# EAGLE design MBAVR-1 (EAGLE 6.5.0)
Minimalistic AVR Board
REV: 123
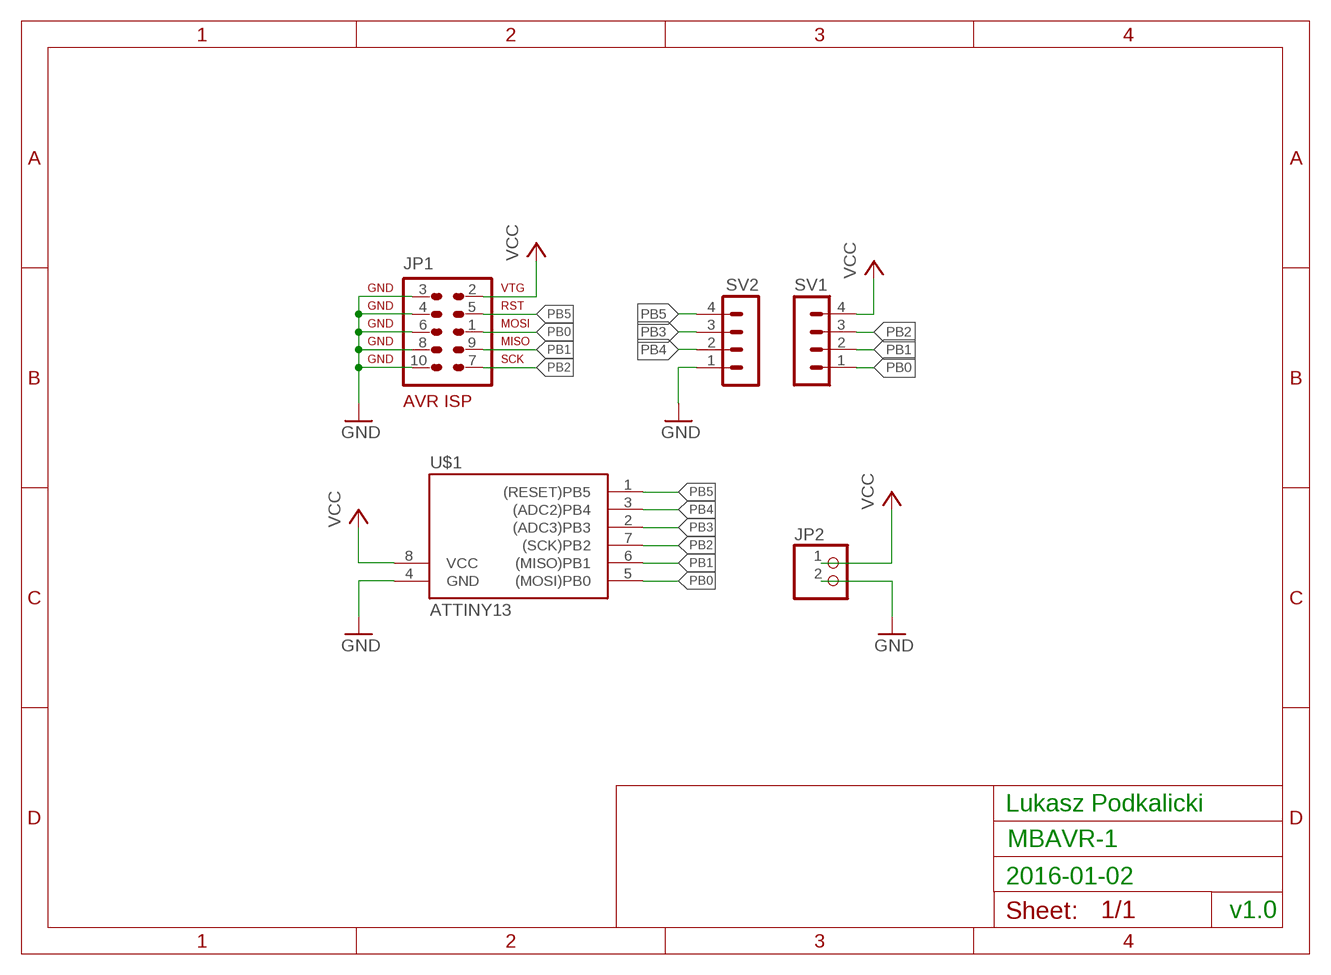
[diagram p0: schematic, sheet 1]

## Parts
JP1  AVR-ISP-10  [AVR-ISP-10]
JP2  PINHD-1X2  [1X02]
SV1  MA04-1  [MA04-1]
SV2  MA04-1  [MA04-1]
U$1  ATTINY13  TINY138P3  [DIL08]

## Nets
GND: JP1.3 JP1.4 JP1.6 JP1.8 JP1.10 JP2.2 SV2.1 U$1.4(GND)
PB0: JP1.1 SV1.1 U$1.5((MOSI)PB0)
PB1: JP1.9 SV1.2 U$1.6((MISO)PB1)
PB2: JP1.7 SV1.3 U$1.7((SCK)PB2)
PB3: SV2.3 U$1.2((ADC3)PB3)
PB4: SV2.2 U$1.3((ADC2)PB4)
PB5: JP1.5 SV2.4 U$1.1((RESET)PB5)
VCC: JP1.2 JP2.1 SV1.4 U$1.8(VCC)

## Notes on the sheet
- Lukasz Podkalicki
- 2016-01-02
- v1.0

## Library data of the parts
JP1 = avr-7:AVR-ISP-10: AVR ISP-10 Serial Programming Header
JP2 = pinhead:PINHD-1X2: PIN HEADER
SV1 SV2 = con-lstb:MA04-1: PIN HEADER; OC_FARNELL: unknown; OC_NEWARK: unknown
U$1 = avr-7:TINY13*

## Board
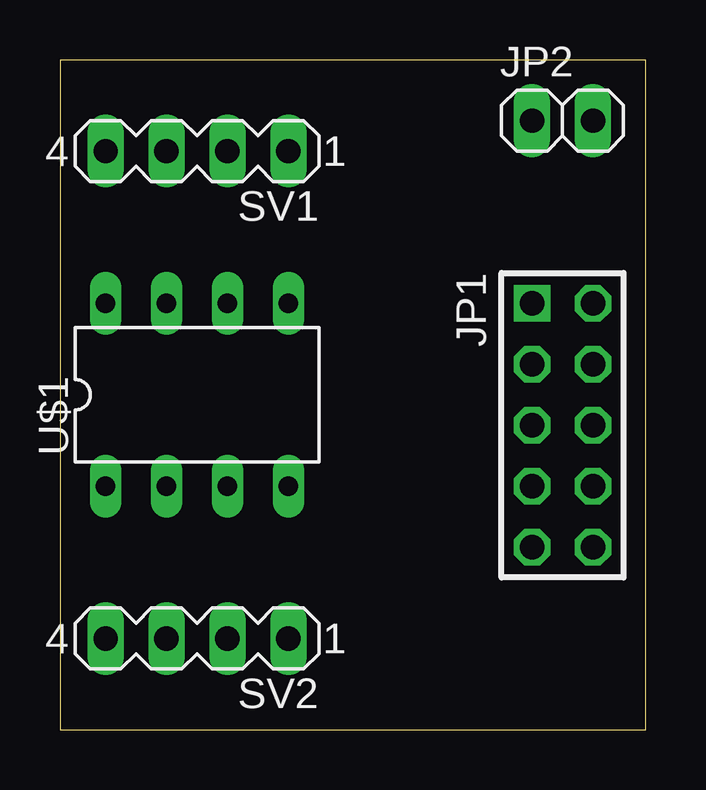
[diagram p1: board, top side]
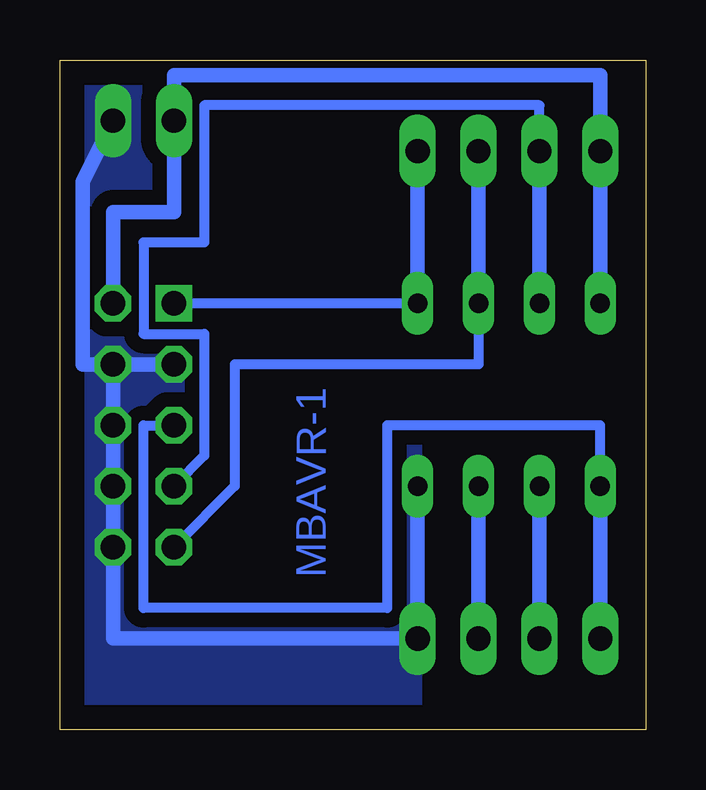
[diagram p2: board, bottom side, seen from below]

Size 24.44 x 27.93 mm. Coordinates in mm from the lower left corner, seen from the top.
Outline: 0,0 24.44,0 24.44,27.93 0,27.93 0,0
Copper layers (1*16): Top 0.035mm / dielectric 1.5mm / Bottom 0.035mm
Design rules "default": minimum track width 10mil, minimum drill 24mil, track to track 8mil, track to pad 8mil, pad to pad 8mil, via to via 8mil, smd to smd 8mil, copper to edge 40mil, drill to drill 8mil, minimum pad ring 10mil, minimum via ring 8mil, stop-mask expansion 4mil, vias tented up to drill 0mil, thermal gap 10mil

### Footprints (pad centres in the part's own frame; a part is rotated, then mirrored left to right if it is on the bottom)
AVR-ISP-10 = drill 1.016 square: 1 -5.08,-1.27 | drill 1.016 octagon: 2 -5.08,1.27; 3 -2.54,-1.27; 4 -2.54,1.27; 5 0,-1.27; 6 0,1.27; 7 2.54,-1.27; 8 2.54,1.27; 9 5.08,-1.27; 10 5.08,1.27
1X02 = drill 1.016 long: 1 -1.27,0; 2 1.27,0
MA04-1 = drill 1.016 long: 1 -3.81,0; 2 -1.27,0; 3 1.27,0; 4 3.81,0
DIL08 = drill 0.813 long: 1 -3.81,-3.81; 2 -1.27,-3.81; 3 1.27,-3.81; 4 3.81,-3.81; 5 3.81,3.81; 6 1.27,3.81; 7 -1.27,3.81; 8 -3.81,3.81

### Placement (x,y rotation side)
JP1  20.95,12.7 270 top
JP2  20.95,25.4 0 top
SV1  5.71,24.13 180 top
SV2  5.71,3.81 180 top
U$1  5.71,13.97 0 top

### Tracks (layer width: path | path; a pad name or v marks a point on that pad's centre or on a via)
GND
  Bottom 0.61: JP1.3 JP1.4 | JP1.4 JP1.6 JP1.8 JP1.10 22.23,3.81 SV2.1 U$1.4 | JP2.2 23.49,22.86 23.49,15.24 JP1.4
  pour Bottom (isolate 0.61, no thermals): 9.52,27.94 24.77,27.94 24.77,0 9.52,0
PB0
  Bottom 0.406: U$1.5 JP1.1
  Bottom 0.61: SV1.1 U$1.5
PB1
  Bottom 0.406: U$1.6 6.98,15.24 17.15,15.24 17.15,10.16 JP1.9
  Bottom 0.61: SV1.2 U$1.6
PB2
  Bottom 0.406: U$1.7 4.45,26.03 18.41,26.03 18.41,20.32 20.95,20.32 20.95,16.51 18.41,16.51 18.41,11.43 JP1.7
  Bottom 0.61: SV1.3 U$1.7
PB3
  Bottom 0.61: SV2.3 U$1.2
PB4
  Bottom 0.61: SV2.2 U$1.3
PB5
  Bottom 0.406: U$1.1 1.91,12.7 10.8,12.7 10.8,5.08 20.95,5.08 20.95,12.7 JP1.5
  Bottom 0.61: SV2.4 U$1.1
VCC
  Bottom 0.61: U$1.8 SV1.4 1.91,27.3 19.69,27.3 JP2.1 19.69,21.59 22.23,21.59 JP1.2

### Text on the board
Bottom: MBAVR-1
_tNames: JP2 | SV1 | JP1 | U$1 | SV2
